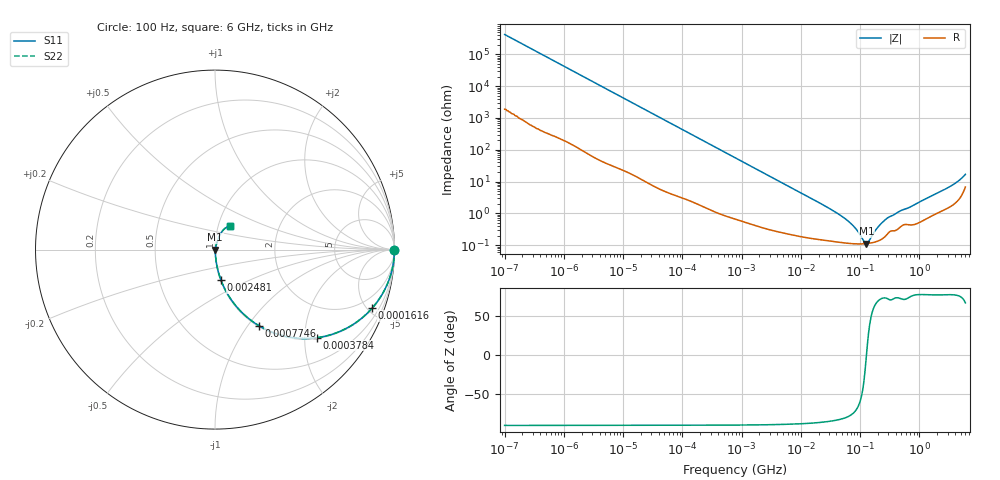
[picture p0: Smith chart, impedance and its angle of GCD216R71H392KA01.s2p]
!Murata Part Number: GCD216R71H392KA01
!These Parameters are Measured in Series Mode Connection
!Data Generated on Jan 08, 2026
!  o--ll--o
!Port1  Port2
!  o------o
!Operation Temp=25[degC], DC Bias Voltage=0[V]
!Freq. Start=100[Hz] Stop=6[GHz] 401[Steps]
# Hz S RI R 50
!Freq.(Hz) S11(Real) S11(Imag) S21(Real) S21(Imag) S12(Real) S12(Imag) S22(Real) S22(Imag)
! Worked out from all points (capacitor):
!   401 points, 100 Hz to 6 GHz, reference 50 ohm
!   read as one part in series: C = 3.74 nF near 109 Hz
!   lowest |Z| = 112 mohm at 127.6 MHz (marker M1)
!   series resonance near 128.3 MHz, so ESL is about 410 pH
!   S11 on the Smith chart (normalised r, x): 100 Hz: open; 161.6 kHz: 1.04, -5.37; 378.4 kHz: 1.02, -2.31; 774.6 kHz: 1.01, -1.13; 2.481 MHz: 1.01, -0.36; 6 GHz: 1.14, +0.31
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100  1 -0.000236  1.1e-06 0.000236  1.1e-06 0.000236  1 -0.000236
2008  1 -0.00469  4.32e-05 0.00469  4.32e-05 0.00469  1 -0.00469
40335  0.9909 -0.0925  0.00914 0.0925  0.00914 0.0925  0.9909 -0.0925
90302  0.9571 -0.1993  0.0429 0.1993  0.0429 0.1993  0.9571 -0.1993
161617  0.8764 -0.3252  0.1236 0.3252  0.1236 0.3252  0.8764 -0.3252
241822  0.7622 -0.4215  0.2378 0.4215  0.2378 0.4215  0.7622 -0.4215
378399  0.5699 -0.4906  0.4301 0.4906  0.4301 0.4906  0.5699 -0.4906
774597  0.2445 -0.424  0.7555 0.424  0.7555 0.424  0.2445 -0.424
1325623  0.1024 -0.296  0.8976 0.296  0.8976 0.296  0.1024 -0.296
2481164  0.0337 -0.1712  0.9663 0.1712  0.9663 0.1712  0.0337 -0.1712
5554849  0.0086 -0.079  0.9914 0.079  0.9914 0.079  0.0086 -0.079
1.555665e7  0.00241 -0.0284  0.9976 0.0284  0.9976 0.0284  0.00241 -0.0284
3.64232e7  0.00142 -0.0115  0.9986 0.0115  0.9986 0.0115  0.00142 -0.0115
5.960426e7  0.00119 -0.00608  0.9988 0.00608  0.9988 0.00608  0.00119 -0.00608
8.154455e7  0.00111 -0.0034  0.9989 0.0034  0.9989 0.0034  0.00111 -0.0034
1.166697e8  0.0011 -0.000697  0.9989 0.000697  0.9989 0.000697  0.0011 -0.000697
1.275994e8  0.00111 -4.15e-05  0.9989 4.15e-05  0.9989 4.15e-05  0.00111 -4.15e-05
1.395531e8  0.00114 0.000617  0.9989 -0.000617  0.9989 -0.000617  0.00114 0.000617
2.088084e8  0.0014 0.00377  0.9986 -0.00377  0.9986 -0.00377  0.0014 0.00377
3.124326e8  0.00264 0.00727  0.9974 -0.00727  0.9974 -0.00727  0.00264 0.00727
2.931063e9  0.0174 0.0582  0.9826 -0.0582  0.9826 -0.0582  0.0174 0.0582
6e9  0.0825 0.1329  0.9175 -0.1329  0.9175 -0.1329  0.0825 0.1329
